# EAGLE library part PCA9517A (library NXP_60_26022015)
Level translating I2C-bus repeater The PCA9517A is a CMOS integrated circuit that provides level shifting between low voltage (down to 0.9 V) and higher voltage (2.7 V to 5.5 V) I2C-bus or SMBus applications. While retaining all the operating modes and features of the I2C-bus system during the level shifts, it also permits extension of the I2C-bus by providing bidirectional buffering for both the data (SDA) and the clock (SCL) lines, thus enabling two buses of 400 pF. Using the PCA9517A enables the system designer to isolate two halves of a bus for both voltage and capacitance. The SDA and SCL pins are overvoltage tolerant and are high-impedance when the PCA9517A is unpowered. The 2.7 V to 5.5 V bus port B drivers behave much like the drivers on the PCA9515A device, while the adjustable voltage bus port A drivers drive more current and eliminate the static offset voltage. This results in a LOW on the port B translating into a nearly 0 V LOW on the port A which accommodates smaller voltage swings of lower voltage logic. The static offset design of the port B PCA9517A I/O drivers prevent them from being connected to another device that has rise time accelerator including the PCA9510, PCA9511, PCA9512, PCA9513, PCA9514, PCA9515A, PCA9516A, PCA9517A (port B), or PCA9518. Port A of two or more PCA9517As can be connected together, however, to allow a star topography with port A on the common bus, and port A can be connected directly to any other buffer with static or dynamic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
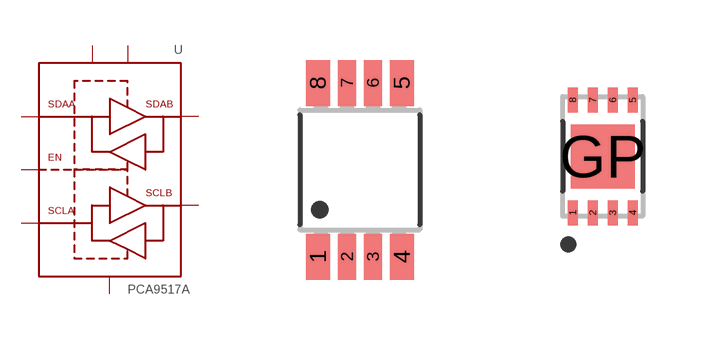
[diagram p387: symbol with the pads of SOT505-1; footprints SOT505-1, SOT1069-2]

Designator prefix U

## PCA9517ADP  [SOT505-1]
1  VCC(A)  pwr
2  SCLA
3  SDAA
4  GND  pwr
5  EN  in
6  SDAB
7  SCLB
8  VCC(B)  pwr

## PCA9517ATP  [SOT1069-2]
1  SDAA
2  GND  pwr
3  EN  in
4  SDAB
5  SCLB
6  VCC(B)  pwr
7  VCC(A)  pwr
8  SCLA

## PCA9517AD  [SOT96-1]
Pads as for SOT505-1

## Footprint SOT505-1 (pad centres in mm)
SOT505-1 TSSOP8: plastic thin shrink small outline package; 8 leads; body width 3 mm JEDEC: -- IEC: --
smd 0.6 x 1.15: 1 -1.05,-2.175; 4 1.05,-2.175; 5 1.05,2.175; 8 -1.05,2.175
smd 0.45 x 1.15: 2 -0.325,-2.175; 3 0.325,-2.175; 6 0.325,2.175; 7 -0.325,2.175

## Footprint SOT1069-2 (pad centres in mm)
SOT1069 HWSON8: plastic thermal enhanced very very thin small outline package; no leads;8 terminals; body 2 x 3 x 0.75 mm JEDEC: IEC: -- JEITA: --
smd 0.25 x 0.625: 1 -0.75,-1.413; 2 -0.25,-1.413; 3 0.25,-1.413; 4 0.75,-1.413; 5 0.75,1.413; 6 0.25,1.413; 7 -0.25,1.413; 8 -0.75,1.413
smd 1.6 x 1.6: GP 0,0

## Footprint SOT96-1 (pad centres in mm)
SOT96-1 SO8: plastic small outline package; 8 leads; body width 3.9 mm JEDEC: MS-012 IEC: 076E03
smd 0.6 x 1.3: 1 -1.905,-2.65; 2 -0.635,-2.65; 3 0.635,-2.65; 4 1.905,-2.65; 5 1.905,2.65; 6 0.635,2.65; 7 -0.635,2.65; 8 -1.905,2.65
